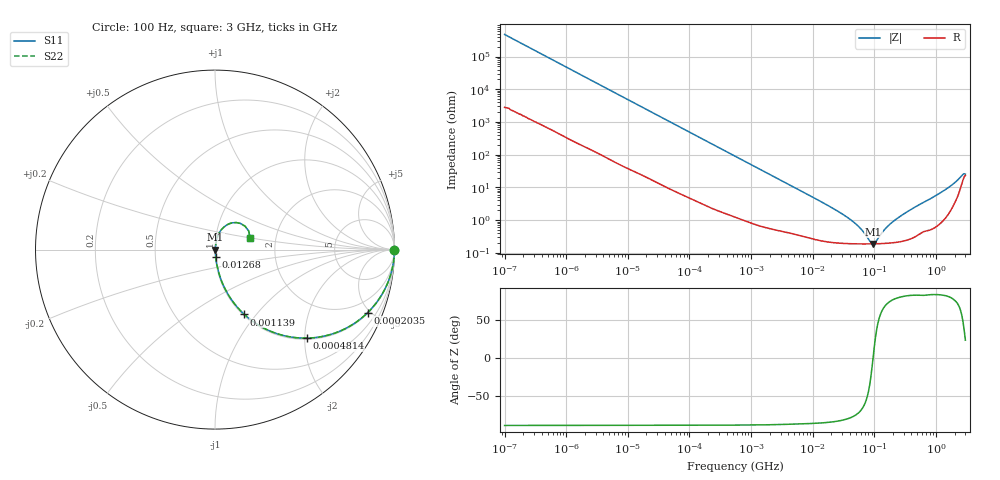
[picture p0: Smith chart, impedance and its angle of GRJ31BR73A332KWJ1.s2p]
!Murata Part Number: GRJ31BR73A332KWJ1
!These Parameters are Measured in Series Mode Connection
!Data Generated on Jun 19, 2026
!  o--ll--o
!Port1  Port2
!  o------o
!Operation Temp=25[degC], DC Bias Voltage=0[V]
!Freq. Start=100[Hz] Stop=3[GHz] 401[Steps]
# Hz S RI R 50
!Freq.(Hz) S11(Real) S11(Imag) S21(Real) S21(Imag) S12(Real) S12(Imag) S22(Real) S22(Imag)
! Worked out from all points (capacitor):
!   401 points, 100 Hz to 3 GHz, reference 50 ohm
!   read as one part in series: C = 3.37 nF near 109 Hz
!   lowest |Z| = 189 mohm at 95.87 MHz (marker M1)
!   series resonance near 95.31 MHz, so ESL is about 830 pH
!   S11 on the Smith chart (normalised r, x): 100 Hz: open; 203.5 kHz: 1.05, -4.81; 481.4 kHz: 1.03, -2.04; 1.139 MHz: 1.01, -0.87; 12.68 MHz: 1.00, -0.08; 3 GHz: 1.47, +0.20
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100  1 -0.000212  1.3e-06 0.000212  1.3e-06 0.000212  1 -0.000212
1788  1 -0.00375  4.1e-05 0.00375  4.1e-05 0.00375  1 -0.00375
31977  0.9951 -0.0657  0.00491 0.0657  0.00491 0.0657  0.9951 -0.0657
97915  0.9595 -0.1925  0.0405 0.1925  0.0405 0.1925  0.9595 -0.1925
203529  0.8498 -0.352  0.1502 0.352  0.1502 0.352  0.8498 -0.352
481374  0.5105 -0.4933  0.4895 0.4933  0.4895 0.4933  0.5105 -0.4933
547723  0.4475 -0.4904  0.5525 0.4904  0.5525 0.4904  0.4475 -0.4904
1138514  0.1632 -0.3611  0.8368 0.3611  0.8368 0.3611  0.1632 -0.3611
2470636  0.0434 -0.1917  0.9566 0.1917  0.9566 0.1917  0.0434 -0.1917
9794414  0.00529 -0.051  0.9947 0.051  0.9947 0.051  0.00529 -0.051
1.268047e7  0.00395 -0.0393  0.9961 0.0393  0.9961 0.0393  0.00395 -0.0393
4.418008e7  0.00198 -0.00908  0.998 0.00908  0.998 0.00908  0.00198 -0.00908
6.234031e7  0.0019 -0.00469  0.9981 0.00469  0.9981 0.00469  0.0019 -0.00469
8.79653e7  0.00188 -0.00086  0.9981 0.00086  0.9981 0.00086  0.00188 -0.00086
9.587315e7  0.00189 6.48e-05  0.9981 -6.48e-05  0.9981 -6.48e-05  0.00189 6.48e-05
1.044919e8  0.00189 0.000991  0.9981 -0.000991  0.9981 -0.000991  0.00189 0.000991
1.412317e8  0.00195 0.00434  0.998 -0.00434  0.998 -0.00434  0.00195 0.00434
1.751444e8  0.00203 0.00695  0.998 -0.00695  0.998 -0.00695  0.00203 0.00695
3.340322e8  0.00273 0.0173  0.9973 -0.0173  0.9973 -0.0173  0.00273 0.0173
1.573002e9  0.0234 0.093  0.9766 -0.093  0.9766 -0.093  0.0234 0.093
2.419119e9  0.0973 0.1494  0.9027 -0.1494  0.9027 -0.1494  0.0973 0.1494
3e9  0.1951 0.0658  0.8049 -0.0658  0.8049 -0.0658  0.1951 0.0658
